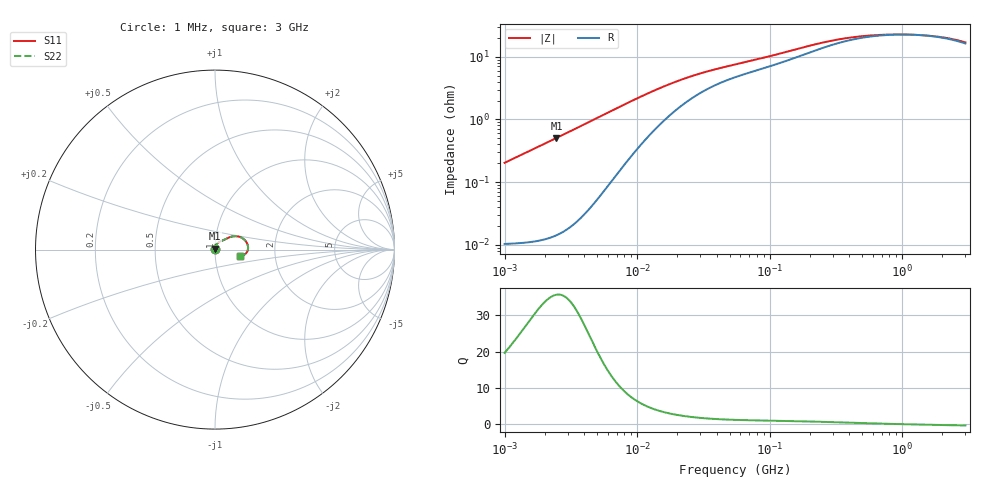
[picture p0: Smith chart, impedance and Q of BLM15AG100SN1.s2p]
! BLM15AG100SN1
# Hz S RI R 50
!Freq.(Hz) S11(Real) S11(Imag) S21(Real) S21(Imag) S12(Real) S12(Imag) S22(Real) S22(Imag)
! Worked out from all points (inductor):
!   401 points, 1 MHz to 3 GHz, reference 50 ohm
!   read as one part in series: L = 32.3 nH near 1.041 MHz
!   highest Q = 35.6 at 2.461 MHz (marker M1), where L = 32.7 nH
!   self-resonance near 1.2 GHz
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1000000  0.000107 0.00203  0.9999 -0.00203  0.9999 -0.00203  0.000107 0.00203
1040844  0.000108 0.00211  0.9999 -0.00211  0.9999 -0.00211  0.000108 0.00211
2461366  0.000167 0.00505  0.9998 -0.00505  0.9998 -0.00505  0.000167 0.00505
3823119  0.000341 0.00796  0.9997 -0.00796  0.9997 -0.00796  0.000341 0.00796
9040831  0.00297 0.0193  0.997 -0.0193  0.997 -0.0193  0.00297 0.0193
1.172775e7  0.00552 0.0246  0.9945 -0.0246  0.9945 -0.0246  0.00552 0.0246
1.461624e7  0.00884 0.0296  0.9912 -0.0296  0.9912 -0.0296  0.00884 0.0296
2.013356e7  0.0159 0.0369  0.9841 -0.0369  0.9841 -0.0369  0.0159 0.0369
2.718395e7  0.0246 0.0431  0.9754 -0.0431  0.9754 -0.0431  0.0246 0.0431
3.74453e7  0.0352 0.0482  0.9648 -0.0482  0.9648 -0.0482  0.0352 0.0482
5.477226e7  0.0479 0.0533  0.9521 -0.0533  0.9521 -0.0533  0.0479 0.0533
8.173662e7  0.0618 0.0599  0.9382 -0.0599  0.9382 -0.0599  0.0618 0.0599
1.148668e8  0.0765 0.0669  0.9235 -0.0669  0.9235 -0.0669  0.0765 0.0669
2.094008e8  0.1141 0.0748  0.8859 -0.0748  0.8859 -0.0748  0.1141 0.0748
2.884452e8  0.1377 0.0707  0.8623 -0.0707  0.8623 -0.0707  0.1377 0.0707
3.973271e8  0.1587 0.0595  0.8413 -0.0595  0.8413 -0.0595  0.1587 0.0595
5.583748e8  0.1745 0.0424  0.8255 -0.0424  0.8255 -0.0424  0.1745 0.0424
8.005644e8  0.1831 0.0223  0.8169 -0.0223  0.8169 -0.0223  0.1831 0.0223
1.171007e9  0.1836 0.00131  0.8164 -0.00131  0.8164 -0.00131  0.1836 0.00131
1.67892e9  0.1757 -0.0169  0.8243 0.0169  0.8243 0.0169  0.1757 -0.0169
2.266846e9  0.1616 -0.029  0.8384 0.029  0.8384 0.029  0.1616 -0.029
3e9  0.1413 -0.0346  0.8587 0.0346  0.8587 0.0346  0.1413 -0.0346
